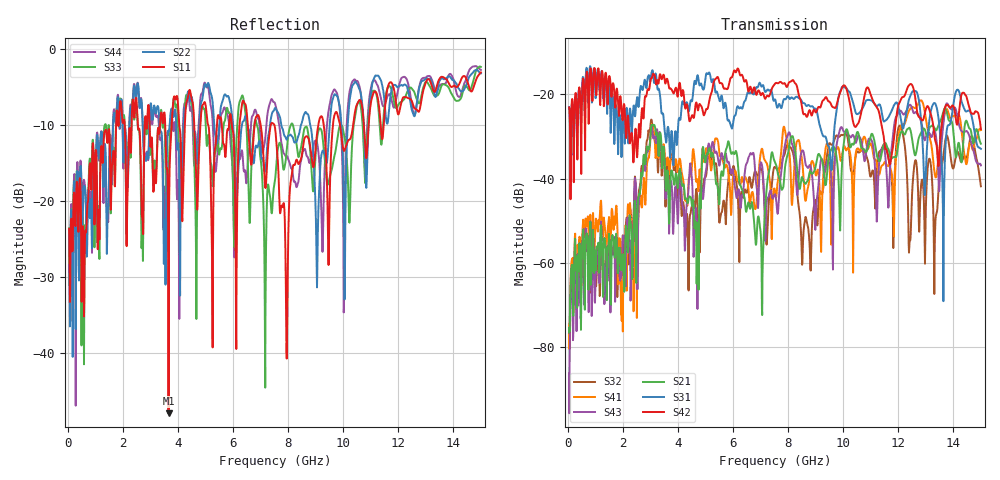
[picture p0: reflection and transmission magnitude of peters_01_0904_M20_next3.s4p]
# MHZ S RI R 50.00
! FREQ  S11  S12  S13  S14
!  S21  S22  S23  S24
!  S31  S32  S33  S34
!  S41  S42  S43  S44
!  REAL  IMAG  REAL  IMAG  REAL  IMAG  REAL  IMAG
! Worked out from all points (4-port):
!   1496 points, 50 MHz to 15 GHz, reference 50 ohm
!   strongest paths, dB at 50 MHz, 3.79 GHz, 7.53 GHz, 11.27 GHz, 15 GHz:
!     S42: -23.1, -19.1, -17.4, -23.6, -28.3
!     S31: -23.1, -29.9, -21.2, -22.6, -33.0
!     S21: -76.6, -38.3, -36.2, -35.4, -31.7
!     S43: -86.3, -43.4, -43.7, -40.3, -36.9
!     S41: -74.9, -34.1, -43.1, -38.3, -28.5
!     S32: -76.0, -35.4, -37.3, -34.6, -41.9
!   lowest |S11| = -47.9 dB at 3.66 GHz (marker M1), VSWR 1.01, Z = 50.4 - j0.0843 ohm
!   |S11| at or under -10 dB: start of sweep to 1.757 GHz; 7.503 GHz to 9.096 GHz (1.594 GHz wide, 19.2 % of centre); 9.886 GHz to 10.36 GHz (476.2 MHz wide, 4.7 % of centre)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
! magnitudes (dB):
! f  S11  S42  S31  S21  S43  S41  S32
! 50 MHz  -23.6  -23.1  -23.1  -76.6  -86.3  -74.9  -76.0
! 1.17 GHz  -19.2  -22.0  -18.7  -57.1  -58.7  -48.0  -67.5
! 2 GHz  -9.7  -26.0  -24.9  -58.3  -54.6  -76.3  -53.5
! 3.09 GHz  -16.2  -15.2  -14.5  -27.2  -29.5  -27.5  -28.1
! 3.66 GHz  -47.9  -17.8  -28.3  -44.2  -44.1  -36.9  -41.7
! 7.05 GHz  -11.3  -19.8  -18.1  -70.7  -36.7  -32.9  -38.0
! 15 GHz  -3.1  -28.3  -33.0  -31.7  -36.9  -28.5  -41.9
